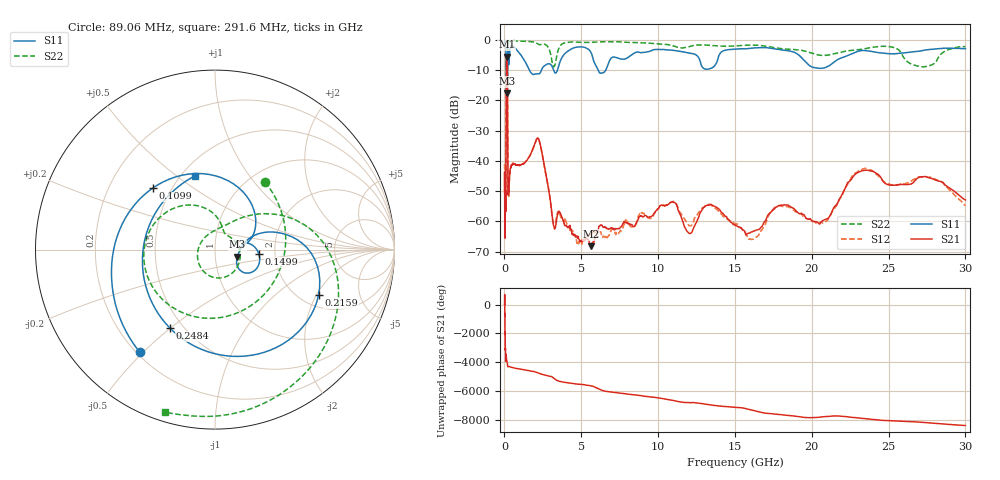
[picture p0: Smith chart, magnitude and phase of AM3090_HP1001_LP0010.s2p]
! Date/Time: Thu, Feb 28, 2019 2:03 PM
! Network Analyzer: Agilent Technologies E8364B Rev: A.07.50.67
! Sweep from 0.010 to 30.000 GHz, 1601 Points, Sweep Type: LOG
! Power Supply: 5.023 V, 0.002 A
# Hz S DB R 50
!freq MagS11 AngS11 MagS21 AngS21 MagS12 AngS12 MagS22 AngS22
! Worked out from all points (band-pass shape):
!   1601 points, 10 MHz to 30 GHz, reference 50 ohm
!   highest |S21| = -5.54 dB at 150.6 MHz (marker M1); lowest = -68.2 dB at 5.64 GHz (marker M2)
!   |S21| within 3 dB of the highest: 123.1 MHz to 187 MHz (63.87 MHz wide, 41.2 % of centre)
!   lowest |S11| = -17.7 dB at 184 MHz (marker M3), VSWR 1.30, Z = 64 - j5.16 ohm
!   |S11| at or under -10 dB: 1.618 GHz to 2.398 GHz (780.1 MHz wide, 38.8 % of centre); 3.206 GHz to 3.449 GHz (242.6 MHz wide, 7.29 % of centre); 6.101 GHz to 6.589 GHz (487.7 MHz wide, 7.69 % of centre)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
!   |S22| runs from -21.2 to -0.2 dB; largest |S21 - S12| = 0.013
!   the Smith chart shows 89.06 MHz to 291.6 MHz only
!   S11 on the Smith chart (normalised r, x): 89.06 MHz: 0.21, -0.49; 109.9 MHz: 0.39, +0.35; 149.9 MHz: 1.64, -0.08; 215.9 MHz: 2.48, -2.08; 248.4 MHz: 0.42, -0.50; 291.6 MHz: 0.58, +0.59
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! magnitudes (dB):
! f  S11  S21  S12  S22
! 10 MHz  -0.2  -50.3  -41.0  -0.5
! 38.04 MHz  -0.5  -61.1  -58.5  -1.3
! 47.89 MHz  -0.7  -50.6  -49.9  -1.5
! 89.06 MHz  -3.0  -50.7  -52.3  -6.6
! 109.9 MHz  -6.2  -20.8  -20.9  -7.9
! 144.7 MHz  -13.2  -5.6  -5.5  -17.7
! 149.9 MHz  -12.2  -5.5  -5.5  -16.5
! 150.6 MHz  -12.1  -5.5  -5.5  -16.4
! 184 MHz  -17.7  -7.8  -7.7  -20.1
! 215.9 MHz  -4.0  -43.1  -43.1  -2.8
! 248.4 MHz  -6.0  -51.0  -50.3  -0.9
! 291.6 MHz  -7.4  -49.2  -49.3  -0.5
! 550.5 MHz  -2.1  -40.8  -40.9  -0.3
! 2.084 GHz  -11.2  -32.9  -32.9  -1.0
! 3.204 GHz  -10.0  -61.3  -60.9  -8.8
! 5.64 GHz  -4.2  -68.2  -63.9  -0.8
! 7.926 GHz  -6.1  -60.5  -59.9  -0.8
! 10.81 GHz  -3.3  -53.6  -53.8  -1.7
! 16.21 GHz  -2.6  -63.1  -65.8  -1.7
! 20.61 GHz  -9.4  -60.1  -60.0  -5.1
! 23.48 GHz  -3.5  -43.1  -42.4  -2.9
! 30 GHz  -2.9  -52.9  -54.8  -2.2
